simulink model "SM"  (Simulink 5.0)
settings: Solver=ode45  StartTime=0.0  StopTime=5  MaxStep=0.001  RelTol=1e-3

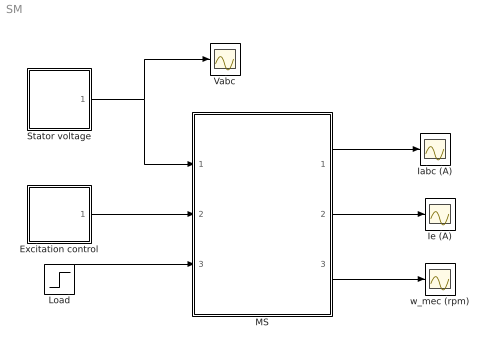
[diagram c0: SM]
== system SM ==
  Excitation control : Subsystem  mask{Ven=63.5, Rex=0.4233, Rex0=4.2, tsinc=1.1, ke=2.294}
  Iabc (A) : Scope
  Ie (A) : Scope
  Load : Step  Time=4  Before=1000  After=20000  SampleTime=0
  MS : Subsystem  mask{p=8, Rs=0.5, Ldm=0.09, Lqm=0.09, Lssig=0.011, LD=0.011, LQ=0.011, LEsig=0.05, LED=0.002, RD=1, RQ=1, Jr=56.095, ke=2.294}
      mask prompts: p "Poles pairs"
      mask init:
      | LEDr=LED/ke; LEsigr=LEsig/(ke^2);
      | Ld=Ldm+[Lssig 0 0; 0 LD+LEDr LEDr; 0 LEDr LEDr+LEsigr]; kd=inv(Ld);
      | Lq=Lqm+[Lssig 0; 0 LQ]; kq=inv(Lq);
      | k=zeros(8,6); k(1,1)=1; k(2,4)=1; k(3,6)=p; k(4:6,1:3)=kd; k(7:8,4:5)=kq;
      | kp1=sqrt(2/3); kp2=1/sqrt(6); kp3=1/sqrt(2);
  Stator voltage : Subsystem  mask{Vn=6000, fn=50, conex='y'}
      mask prompts: Vn "V1 (V) -line rms voltage"; fn "f1 (Hz)"; conex "Winding conexion ('y' or 'd')"
      mask init:
      | if strcmp(lower(conex),'y')
      | Vm=Vn*sqrt(2/3);
      | else
      | Vm=Vn*sqrt(2);
      | end
      | wn=2*pi*fn;
  Vabc : Scope
  w_mec (rpm) : Scope
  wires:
  MS/1(Iabc) -> Iabc (A)/1
  Excitation control/1(VexRex) -> MS/2(Ex)
  Load/1 -> MS/3(Tload)
  Stator voltage/1(Vabc) -> MS/1(Vabc), Vabc/1
  MS/2(Ie) -> Ie (A)/1
  MS/3(wmec) -> w_mec (rpm)/1

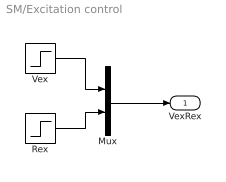
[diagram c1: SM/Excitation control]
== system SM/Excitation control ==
  Mux : Mux  Inputs=2
  Rex : Step  Time=tsinc  Before=Rex0/ke^2  After=Rex/ke^2  SampleTime=0
  Vex : Step  Time=tsinc  After=Ven/ke  SampleTime=0
  VexRex : Outport
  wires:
  Rex/1 -> Mux/2
  Vex/1 -> Mux/1
  Mux/1 -> VexRex/1

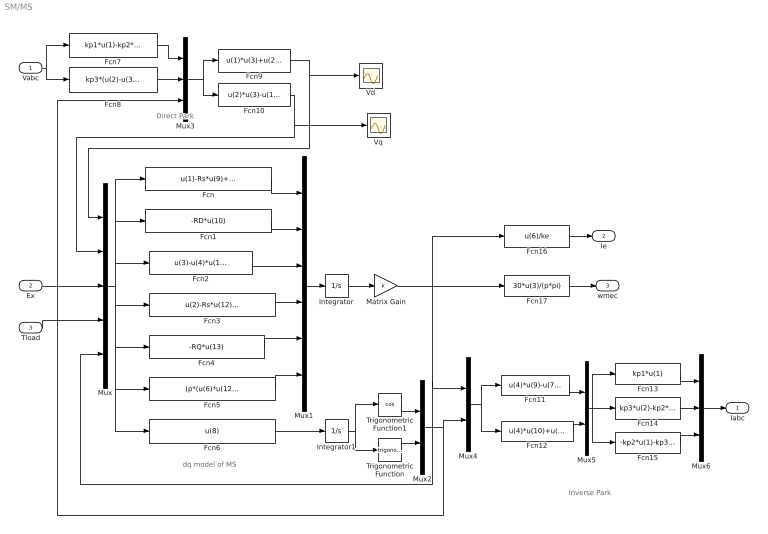
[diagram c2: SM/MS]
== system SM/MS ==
  note: Inverse Park
  note: Direct Park
  note: dq model of MS
  Vabc : Inport
  Ex : Inport  Port=2
  Tload : Inport  Port=3
  Fcn : Fcn  Expr=u(1)-Rs*u(9)+u(8)*u(7)
  Fcn1 : Fcn  Expr=-RD*u(10)
  Fcn10 : Fcn  Expr=u(2)*u(3)-u(1)*u(4)
  Fcn11 : Fcn  Expr=u(4)*u(9)-u(7)*u(10)
  Fcn12 : Fcn  Expr=u(4)*u(10)+u(7)*u(9)
  Fcn13 : Fcn  Expr=kp1*u(1)
  Fcn14 : Fcn  Expr=kp3*u(2)-kp2*u(1)
  Fcn15 : Fcn  Expr=-kp2*u(1)-kp3*u(2)
  Fcn16 : Fcn  Expr=u(6)/ke
  Fcn17 : Fcn  Expr=30*u(3)/(p*pi)
  Fcn2 : Fcn  Expr=u(3)-u(4)*u(11)
  Fcn3 : Fcn  Expr=u(2)-Rs*u(12)-u(8)*u(6)
  Fcn4 : Fcn  Expr=-RQ*u(13)
  Fcn5 : Fcn  Expr=(p*(u(6)*u(12)-u(7)*u(9))-u(5))/Jr
  Fcn6 : Fcn  Expr=u(8)
  Fcn7 : Fcn  Expr=kp1*u(1)-kp2*(u(2)+u(3))
  Fcn8 : Fcn  Expr=kp3*(u(2)-u(3))
  Fcn9 : Fcn  Expr=u(1)*u(3)+u(2)*u(4)
  Integrator : Integrator
  Integrator1 : Integrator
  Matrix Gain : Gain  Gain=k  Multiplication=Matrix(K*u)
  Mux : Mux  Inputs=5
  Mux1 : Mux  Inputs=6
  Mux2 : Mux  Inputs=2
  Mux3 : Mux  Inputs=3
  Mux4 : Mux  Inputs=2
  Mux5 : Mux  Inputs=2
  Mux6 : Mux  Inputs=3
  Trigonometric Function : Trigonometry
  Trigonometric Function1 : Trigonometry  Operator=cos
  Vd : Scope
  Vq : Scope
  Iabc : Outport
  Ie : Outport  Port=2
  wmec : Outport  Port=3
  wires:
  Mux/1 -> Fcn4/1, Fcn5/1, Fcn6/1, Fcn3/1, Fcn/1, Fcn1/1, Fcn2/1
  Ex/1 -> Mux/3
  Fcn/1 -> Mux1/1
  Fcn1/1 -> Mux1/2
  Fcn2/1 -> Mux1/3
  Fcn3/1 -> Mux1/4
  Fcn4/1 -> Mux1/5
  Mux1/1 -> Integrator/1
  Integrator1/1 -> Trigonometric Function/1, Trigonometric Function1/1
  Trigonometric Function1/1 -> Mux2/1
  Trigonometric Function/1 -> Mux2/2
  Mux2/1 -> Mux4/2, Mux3/3
  Fcn11/1 -> Mux5/1
  Fcn12/1 -> Mux5/2
  Mux5/1 -> Fcn14/1, Fcn15/1, Fcn13/1
  Fcn13/1 -> Mux6/1
  Fcn14/1 -> Mux6/2
  Fcn15/1 -> Mux6/3
  Mux6/1 -> Iabc/1
  Tload/1 -> Mux/4
  Vabc/1 -> Fcn7/1, Fcn8/1
  Fcn7/1 -> Mux3/1
  Fcn8/1 -> Mux3/2
  Fcn10/1 -> Mux/2, Vq/1
  Fcn9/1 -> Vd/1, Mux/1
  Fcn6/1 -> Integrator1/1
  Fcn5/1 -> Mux1/6
  Mux4/1 -> Fcn11/1, Fcn12/1
  Mux3/1 -> Fcn9/1, Fcn10/1
  Integrator/1 -> Matrix Gain/1
  Matrix Gain/1 -> Mux4/1, Mux/5, Fcn16/1, Fcn17/1
  Fcn16/1 -> Ie/1
  Fcn17/1 -> wmec/1

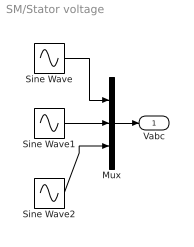
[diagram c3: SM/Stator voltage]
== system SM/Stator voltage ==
  Mux : Mux  Inputs=3
  Sine Wave : Sin  Amplitude=Vm  Frequency=wn  SampleTime=0
  Sine Wave1 : Sin  Amplitude=Vm  Frequency=wn  Phase=-2*pi/3  SampleTime=0
  Sine Wave2 : Sin  Amplitude=Vm  Frequency=wn  Phase=2*pi/3  SampleTime=0
  Vabc : Outport
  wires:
  Sine Wave1/1 -> Mux/2
  Sine Wave2/1 -> Mux/3
  Sine Wave/1 -> Mux/1
  Mux/1 -> Vabc/1
